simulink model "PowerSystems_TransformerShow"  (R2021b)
settings: Solver=VariableStepAuto  StartTime=0.0  StopTime=60e-3  RelTol=1e-3
libraries: spsGroundLib x1, spsMutualInductanceLib x1, eeTransforms x1, spsThreePhaseSeriesRLCBranchLib x1, spsThreePhaseVIMeasurementLib x1, spsThreePhaseSourceLib x1, spspowerguiLib x1

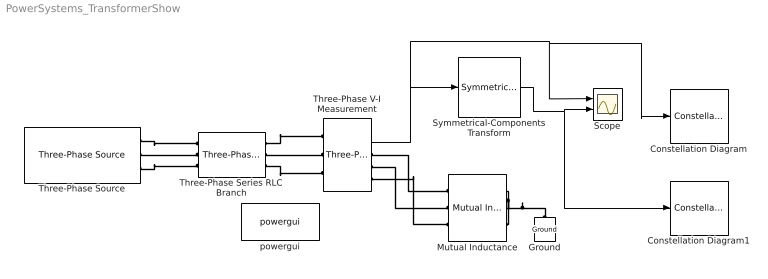
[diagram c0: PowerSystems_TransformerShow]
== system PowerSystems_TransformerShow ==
  Constellation Diagram : ConstellationDiagram
  Constellation Diagram1 : ConstellationDiagram
  Ground : spsGroundLib/Ground  LConnTagsString=a
  Mutual Inductance : spsMutualInductanceLib/Mutual Inductance  LConnTagsString=a|b|c  RConnTagsString=A|B|C  TypeOfMutual=Two or three windings with equal mutual terms  NumberOfWindings=3  SelfImpedance1=[1.1 1.1e-03]  SelfImpedance2=[ 1.1 1.1e-03]  ThreeWindings=on  SelfImpedance3=[ 1.1 1.1e-03]  MutualImpedance=[1.0 1.0e-03]  InductanceMatrix="[1.0 0.9  0.9 ;  0.9 1.0  0.9;  0.9 0.9 1.0 ] * 1e-3"  ResistanceMatrix="[1.0 0.9  0.9 ;  0.9 1.0  0.9;  0.9 0.9 1.0 ]"  Measurements=None
  Scope : Scope  NumInputPorts=2
  Symmetrical-Components Transform : eeTransforms/Symmetrical-Components Transform  PowerInvariant=off
  Three-Phase Series RLC Branch : spsThreePhaseSeriesRLCBranchLib/Three-Phase Series RLC Branch  LConnTagsString=A|B|C  RConnTagsString=A|B|C  BranchType=R  Resistance=10  Inductance=0  Capacitance=0  Measurements=None
  Three-Phase V-I Measurement : spsThreePhaseVIMeasurementLib/Three-Phase V-I Measurement  VoltageMeasurement=phase-to-ground  SetLabelV=off  LabelV=Vabc  Vpu=off  VpuLL=off  CurrentMeasurement=yes  SetLabelI=off  LabelI=Iabc  Ipu=off  Pbase=100e6  Vbase=500e3  OutputType=Complex  PhasorSimulation=on  PSBequivalent=0
  Three-Phase Source : spsThreePhaseSourceLib/Three-Phase Source  InternalConnection=Yg  VoltagePhases=off  Voltage=380  PhaseAngle=0  Voltage_phases=[25e3 25e3 25e3]/sqrt(3)  PhaseAngles_phases=[0 -120 +120]  Frequency=50  NonIdealSource=on  SpecifyImpedance=off  Resistance=0  Inductance=0  ShortCircuitLevel=100e6  BaseVoltage=380  XRratio=7  BusType=swing  Pref=10e3  Qref=0  Prefabc=[10e3, 10e3, 10e3]  Qrefabc=[0, 0, 0]  Qmin=-inf  Qmax=inf
  powergui : spspowerguiLib/powergui  Priority=1  SimulationMode=Discrete phasor  SampleTime=50e-6  frequency=50  Iterations=50  frequencyindice=50  Pbase=100e6  ErrMax=1e-4  UnitsV=kV  UnitsW=MW  buscounter=0  FunctionMessages=off  echomessages=off  EnableUseOfTLC=off  CurrentSourceSwitches=off  DisableSnubberDevices=off  DisableRonSwitches=off  DisableVfSwitches=off  DisplayEquations=off  AutomaticDiscreteSolvers=off  SolverType=Tustin/Backward Euler (TBE)  Interpol=off  ExternalGateDelay=off  methode=off  Ts=100  x0status=blocks  SPID=on  SwTol=0  HookPort=off  NonlinearTolerance=1e-4  nMaxIteration=100  ContinueOnMaxIteration=off  RestoreLinks=warning  ResistiveCurrentMeasurement=off  Frange=[0:2:500]  Ylog=off  Xlog=on  ShowGrid=off  save=off  variable=ZData  structure=0  ZoomFFT=off  StartTime=0.0  cycles=1  DisplayStyle=1  fundamental=60  FreqAxis=off  MaxFrequency=1000  frequencyindicesteady=1  RmsSteady=1  display=off
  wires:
  Symmetrical-Components Transform/1 -> Constellation Diagram1/1, Scope/2
  Three-Phase V-I Measurement/2 -> Constellation Diagram/1, Scope/1, Symmetrical-Components Transform/1
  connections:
  Three-Phase Source/RConn1 -- Three-Phase Series RLC Branch/LConn1
  Three-Phase Source/RConn2 -- Three-Phase Series RLC Branch/LConn2
  Three-Phase Source/RConn3 -- Three-Phase Series RLC Branch/LConn3
  Three-Phase Series RLC Branch/RConn1 -- Three-Phase V-I Measurement/LConn1
  Three-Phase Series RLC Branch/RConn2 -- Three-Phase V-I Measurement/LConn2
  Three-Phase Series RLC Branch/RConn3 -- Three-Phase V-I Measurement/LConn3
  Three-Phase V-I Measurement/RConn1 -- Mutual Inductance/LConn1
  Three-Phase V-I Measurement/RConn2 -- Mutual Inductance/LConn2
  Mutual Inductance/LConn3 -- Three-Phase V-I Measurement/RConn3
  Mutual Inductance/RConn3 -- Mutual Inductance/RConn2 -- Mutual Inductance/RConn1 -- Ground/LConn1
